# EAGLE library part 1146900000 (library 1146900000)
PCB plug-in connector, male header, open side, THT solder connection, 5.08 mm, Number of poles: 10, 90, Solder pin length: 3.2 mm, tinned, orange, Box Source: Datasheet
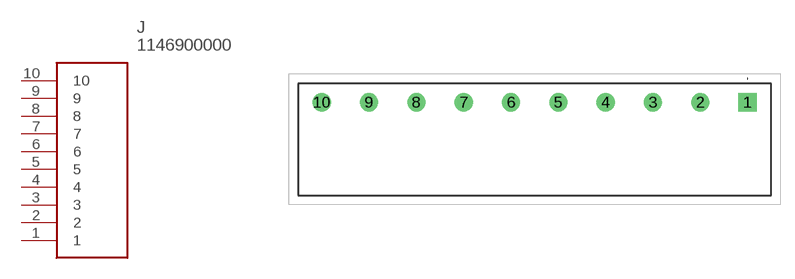
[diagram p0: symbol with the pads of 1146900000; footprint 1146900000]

Designator prefix J

## 1146900000 (Description: PCB plug-in connector, male header, open side, THT solder connection, 5.08 mm, Number of poles: 10, 90, Solder pin length: 3.2 mm, tinned, orange, Box; Height: 8.4mm; Manufacturer_Name: Weidmuller; Manufacturer_Part_Number: 1146900000)  [1146900000]
1  1
2  2
3  3
4  4
5  5
6  6
7  7
8  8
9  9
10  10

## Footprint 1146900000 (pad centres in mm)
1146900000-1
drill 1.3 pad 1.95 square: 1 0,0
drill 1.3 pad 1.95: 2 -5.08,0; 3 -10.16,0; 4 -15.24,0; 5 -20.32,0; 6 -25.4,0; 7 -30.48,0; 8 -35.56,0; 9 -40.64,0; 10 -45.72,0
